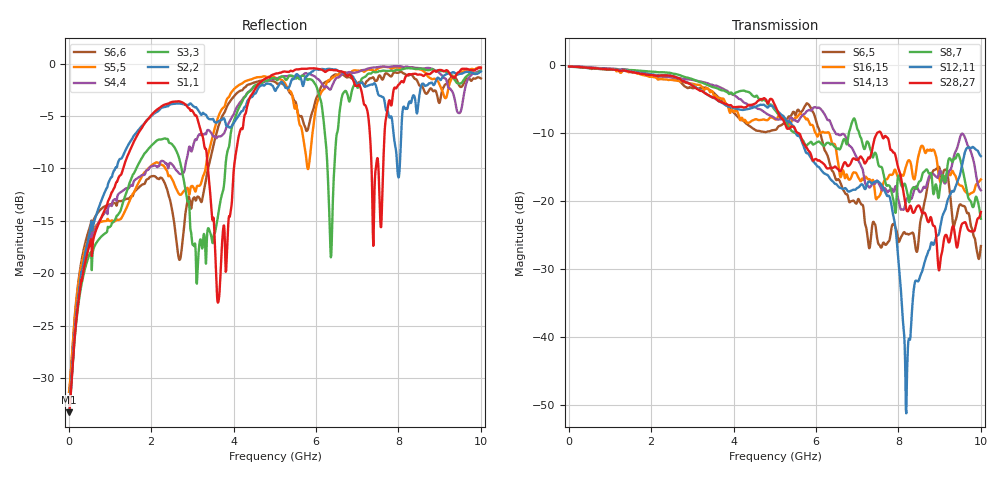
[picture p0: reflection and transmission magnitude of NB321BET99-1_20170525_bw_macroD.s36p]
! Touchstone(R) file created by SIwave 2017.0.0
! Touchstone(R) file created on Mon Jun 05 11:37:27 2017
! Port[1] = D_DN_0__DIE_189
! Port[2] = D_DN_0__LGA_AK22
! Port[3] = D_DN_1__DIE_193
! Port[4] = D_DN_1__LGA_AK24
! Port[5] = D_DN_2__DIE_197
! Port[6] = D_DN_2__LGA_AL27
! Port[7] = D_DN_3__DIE_203
! Port[8] = D_DN_3__LGA_U31
! Port[9] = D_DN_4__DIE_213
! Port[10] = D_DN_4__LGA_AE31
! Port[11] = D_DN_5__DIE_219
! Port[12] = D_DN_5__LGA_Y30
! Port[13] = D_DN_6__DIE_223
! Port[14] = D_DN_6__LGA_AA31
! Port[15] = D_DN_7__DIE_227
! Port[16] = D_DN_7__LGA_AC31
! Port[17] = D_DP_0__DIE_190
! Port[18] = D_DP_0__LGA_AL23
! Port[19] = D_DP_1__DIE_194
! Port[20] = D_DP_1__LGA_AL25
! Port[21] = D_DP_2__DIE_198
! Port[22] = D_DP_2__LGA_AK26
! Port[23] = D_DP_3__DIE_204
! Port[24] = D_DP_3__LGA_V30
! Port[25] = D_DP_4__DIE_214
! Port[26] = D_DP_4__LGA_AF30
! Port[27] = D_DP_5__DIE_220
! Port[28] = D_DP_5__LGA_W31
! Port[29] = D_DP_6__DIE_224
! Port[30] = D_DP_6__LGA_AB30
! Port[31] = D_DP_7__DIE_228
! Port[32] = D_DP_7__LGA_AD30
! Port[33] = DCLK_DN_DIE_208
! Port[34] = DCLK_DN_LGA_AH30
! Port[35] = DCLK_DP_DIE_209
! Port[36] = DCLK_DP_LGA_AG31
! S-parameters (magnitude in dB)
# Hz S DB R 50.000000
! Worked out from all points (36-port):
!   1000 points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, 10 MHz to 10 GHz, reference 50 ohm
!   strongest paths, dB at 10 MHz, 2.51 GHz, 5.01 GHz, 7.51 GHz, 10 GHz:
!     S28,27: -0.3, -1.7, -6.0, -9.9, -21.6
!     S12,11: -0.3, -1.7, -6.4, -17.2, -13.4
!     S8,7: -0.3, -1.3, -6.7, -14.6, -22.6
!     S14,13: -0.2, -1.9, -7.9, -17.4, -18.4
!     S16,15: -0.2, -2.2, -8.0, -19.5, -16.9
!     S6,5: -0.2, -1.9, -9.6, -26.3, -26.6
!   lowest |S11| = -33.3 dB at 10 MHz (marker M1), VSWR 1.04, Z = 52.2 + j0.311 ohm
!   |S11| at or under -10 dB: start of sweep to 1.323 GHz; 3.377 GHz to 4.008 GHz (630.9 MHz wide, 17.1 % of centre); 7.514 GHz to 7.629 GHz (114.7 MHz wide, 1.51 % of centre)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
